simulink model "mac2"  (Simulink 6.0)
settings: Solver=ode45  StartTime=0.0  StopTime=2000  RelTol=1e-3
undefined symbols (not defined in the file or in its folder): coef, data, Ft, netlist, Ts
libraries: xbsIndex_r3 x35, dspsnks4 x1

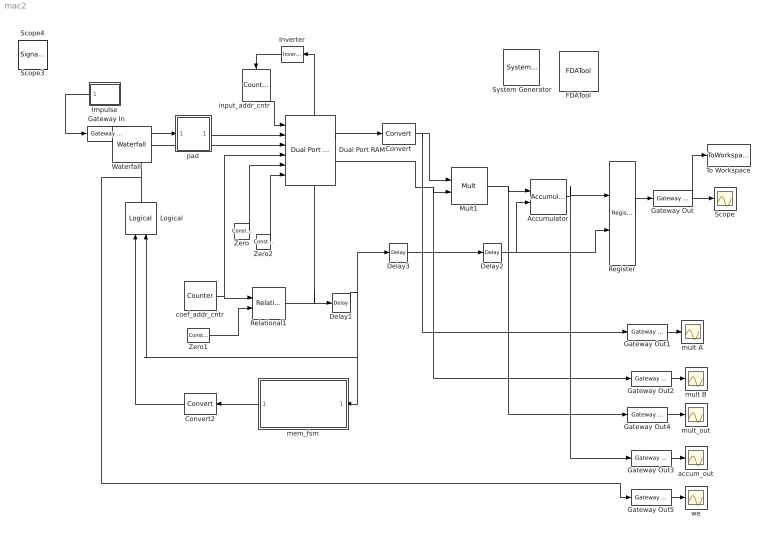
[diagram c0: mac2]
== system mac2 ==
  " System Generator" : xbsIndex_r3/ System Generator  Tag=genX  xilinxfamily=Virtex2  part=xc2v1000  speed=-4  package=fg456  synthesis_tool=XST  directory=./netlist  testbench=off  simulink_period=1/2  sysclk_period=10  incr_netlist=off  trim_vbits=Everywhere in SubSystem  dbl_ovrd=According to Block Masks  core_generation=According to Block Masks  run_coregen=off  deprecated_control=off  eval_field=0
  Accumulator : xbsIndex_r3/Accumulator  n_bits=26  overflow=Wrap  operation=Add  scale=1  explicit_period=on  period=1  rst=on  hasbypass=off  en=off  dbl_ovrd=off  show_param=off  gen_core=off  use_rpm=on
  Convert : xbsIndex_r3/Convert  arith_type=Unsigned  n_bits=8  bin_pt=6  quantization=Truncate  overflow=Wrap  latency=0  explicit_period=off  period=1  dbl_ovrd=off  show_param=off  inserted_by_tool=off  pipeline=off
  Convert2 : xbsIndex_r3/Convert  Orientation=left  arith_type=Boolean  n_bits=8  bin_pt=6  quantization=Truncate  overflow=Wrap  latency=0  explicit_period=off  period=1  dbl_ovrd=off  show_param=off  inserted_by_tool=off  pipeline=off
  Delay1 : xbsIndex_r3/Delay  latency=1  reg_retiming=off  explicit_period=off  period=1  en=off  accept_only_valid=off  init_zero=on  dbl_ovrd=off  show_param=off
  Delay2 : xbsIndex_r3/Delay  latency=3  reg_retiming=off  explicit_period=off  period=1  en=off  accept_only_valid=off  init_zero=on  dbl_ovrd=off  show_param=off
  Delay3 : xbsIndex_r3/Delay  latency=1  reg_retiming=off  explicit_period=off  period=1  en=off  accept_only_valid=off  init_zero=on  dbl_ovrd=off  show_param=off
  Dual Port RAM1 : xbsIndex_r3/Dual Port RAM  depth=length(coef)*2  initVector=[ (data) (coef)]  write_mode_A=Read After Write  write_mode_B=Read After Write  latency=1  mem_collision=off  init_zero=on  explicit_period=off  period=1  dbl_ovrd=off  rst_a=off  init_a=0  rst_b=off  init_b=0  show_param=off  distributed_mem=off  use_rpm=off  gen_core=off
  FDATool : xbsIndex_r3/FDATool
  Gateway In : xbsIndex_r3/Gateway In  arith_type=Unsigned  n_bits=8  bin_pt=6  quantization=Truncate  overflow=Wrap  period=1  timing_constraint=None  locs_specified=off  LOCs={}  needs_fixed_name=off  dbl_ovrd=off  show_param=off
  Gateway Out{,1..5} (6 alike) : xbsIndex_r3/Gateway Out  output_type=Double  nbits=8  bin_pt=6  arith_type=Boolean  quantization=Truncate  overflow=Wrap  hdl_port=on  timing_constraint=None  locs_specified=off  LOCs={}  needs_fixed_name=off  show_param=off
  Impulse : Subsystem  Orientation=left
  Inverter : xbsIndex_r3/Inverter  Orientation=left  latency=0  explicit_period=off  period=1  en=off  dbl_ovrd=off  show_param=off
  Logical : xbsIndex_r3/Logical  Orientation=up  logical_function=AND  inputs=2  precision=Full  arith_type=Unsigned  n_bits=0  bin_pt=0  align_bp=on  latency=0  explicit_period=off  period=1  en=off  dbl_ovrd=off  show_param=off
  Mult1 : xbsIndex_r3/Mult  precision=User Defined  arith_type="Signed  (2's comp)"  n_bits=26  bin_pt=17  quantization=Truncate  overflow=Wrap  latency=3  explicit_period=off  period=1  en=off  dbl_ovrd=off  show_param=off  mult_type=Parallel  oversample=2  use_embedded=off  pipeline=on  use_rpm=on  placement_style=Rectangular Shape  gen_core=off
  Register : xbsIndex_r3/Register  init=0  reg_only_valid=on  explicit_period=off  period=1  rst=off  en=on  out_en=off  dbl_ovrd=off  show_param=off
  Relational1 : xbsIndex_r3/Relational  mode=a=b  latency=0  explicit_period=on  period=-1  en=off  dbl_ovrd=off  show_param=off
  Scope : Scope
  To Workspace : ToWorkspace  VariableName=simout  SampleTime=-1  SaveFormat=Array
  Zero : xbsIndex_r3/Constant  Priority=5  const=0  equ=P=C  arith_type="Signed  (2's comp)"  n_bits=12  bin_pt=11  opselect=C  inp2=PCIN>>17  opr=+  inp1=P  carry=CIN  iostate=0  explicit_period=on  period=1  dbl_ovrd=off
  Zero1 : xbsIndex_r3/Constant  Priority=5  const=63  equ=P=C  arith_type=Unsigned  n_bits=2*log2(length(coef))  bin_pt=0  opselect=C  inp2=PCIN>>17  opr=+  inp1=P  carry=CIN  iostate=0  explicit_period=off  period=1  dbl_ovrd=off
  Zero2 : xbsIndex_r3/Constant  Priority=5  const=0  equ=P=C  arith_type=Boolean  n_bits=12  bin_pt=11  opselect=C  inp2=PCIN>>17  opr=+  inp1=P  carry=CIN  iostate=0  explicit_period=off  period=1/8000  dbl_ovrd=off
  accum_out : Scope
  coef_addr_cntr : xbsIndex_r3/Counter  Priority=5  cnt_type=Count Limited  n_bits=ceil(log2(2*length(coef)))  bin_pt=0  arith_type=Unsigned  start_count=32  cnt_to=63  cnt_by_val=1  operation=Up  explicit_period=off  period=1  load_pin=off  rst=off  en=off  dbl_ovrd=off  show_param=off  use_rpm=on  gen_core=on
  input_addr_cntr : xbsIndex_r3/Counter  Orientation=down  Priority=5  cnt_type=Count Limited  n_bits=ceil(log2(2*length(coef)))  bin_pt=0  arith_type=Unsigned  start_count=0  cnt_to=31  cnt_by_val=1  operation=Up  explicit_period=off  period=1/8000  load_pin=off  rst=off  en=on  dbl_ovrd=off  show_param=off  use_rpm=on  gen_core=on
  mem_fsm : Subsystem  Orientation=left
  mult A : Scope
  mult B : Scope
  mult_out : Scope
  pad : Subsystem
  we : Scope
  Scope3 : SignalViewerScope  IOType=viewer  RefreshTime=0.035000
  Scope4 : SignalViewerScope  IOType=viewer  RefreshTime=0.035000
  Waterfall : dspsnks4/Waterfall  IOType=viewer  TraceProperties=off  NumTraces=6  CMapStr=autumn  TNewest=1  TOldest=0  HistoryLength=10  HistoryFull=Overwrite  UpdateInterval=1  ExportMode=Selected  MLExportName=ExportData  AutoExport=off  DisplayProperties=off  MouseMode=Orbit  AxisGrid=on  Snapshot=off  Suspend=off  SyncSnapshots=off  OpenScopeAtSimStart=off  FigPos=[243 195 405 320]  CameraView=[69.4600750684385 564.426060114276 -133.474523953492 0 18.5 3.5 0.616338299486424 -7.9078811427274 1.98411164834144 2.40985953613679 1 18.5 3]  InportDimsHint=[32 1]  AxisProperties=off  AxisColor='w'  XLabel=Amplitude  YLabel=Samples  ZLabel=Time  TriggerProperties=off  TrigStartMode=Immediately  TrigStartT=0  TrigStartN=0  TrigStartFcn=trigbegin  TrigStopMode=Never  TrigStopT=0.1  TrigStopN=1  TrigStopFcn=trigend  TrigRearmMode=Never  TrigRearmT=0  TrigRearmN=0  TrigRearmFcn=trigrearm  XformProperties=on  XformMode=None  XformFcn=abs  XformExpr=(u+1)/2
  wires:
  Gateway Out/1 -> Scope/1, To Workspace/1
  Impulse/1(Out1) -> Gateway In/1
  Mult1/1 -> Accumulator/1, Gateway Out4/1
  Zero1/1 -> Relational1/2
  input_addr_cntr/1 -> Dual Port RAM1/1
  Dual Port RAM1/2 -> Mult1/2, Gateway Out2/1
  Inverter/1 -> input_addr_cntr/1
  Zero/1 -> Dual Port RAM1/5
  Zero2/1 -> Dual Port RAM1/6
  Delay2/1 -> Accumulator/2, Register/2
  Delay3/1 -> Delay2/1
  Relational1/1 -> Inverter/1, Delay1/1
  Accumulator/1 -> Register/1, Gateway Out3/1
  Register/1 -> Gateway Out/1
  Dual Port RAM1/1 -> Convert/1
  Convert/1 -> Mult1/1, Gateway Out1/1
  Gateway Out1/1 -> mult A/1
  Gateway Out2/1 -> mult B/1
  Gateway Out4/1 -> mult_out/1
  Delay1/1 -> Delay3/1, Logical/2, mem_fsm/1(fsm_cntr_in)
  mem_fsm/1(fsm_we_out) -> Convert2/1
  Logical/1 -> Dual Port RAM1/3, Gateway Out5/1
  Convert2/1 -> Logical/1
  coef_addr_cntr/1 -> Relational1/1, Dual Port RAM1/4
  pad/1(Out1) -> Dual Port RAM1/2
  Gateway In/1 -> pad/1(In1)
  Gateway Out5/1 -> we/1
  Gateway Out3/1 -> accum_out/1

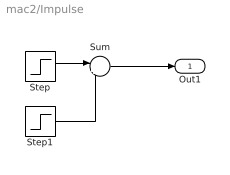
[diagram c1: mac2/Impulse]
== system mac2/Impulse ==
  Step : Step  Time=1*Ts  SampleTime=Ts
  Step1 : Step  Time=2*Ts  SampleTime=Ts
  Sum : Sum  Inputs=|+-
  Out1 : Outport
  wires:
  Step/1 -> Sum/1
  Sum/1 -> Out1/1
  Step1/1 -> Sum/2

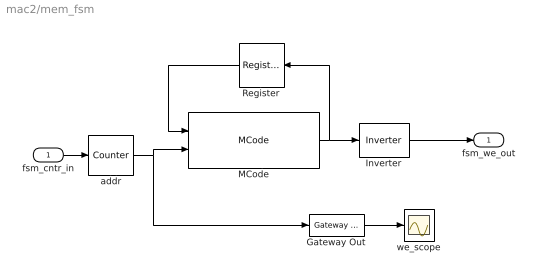
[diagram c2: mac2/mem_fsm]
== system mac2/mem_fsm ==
  fsm_cntr_in : Inport  Port=1  LatchInput=off
  Gateway Out : xbsIndex_r3/Gateway Out  output_type=Double  nbits=8  bin_pt=6  arith_type=Boolean  quantization=Truncate  overflow=Wrap  hdl_port=on  timing_constraint=None  locs_specified=off  LOCs={}  needs_fixed_name=off  show_param=off
  Inverter : xbsIndex_r3/Inverter  latency=0  explicit_period=off  period=1  en=off  dbl_ovrd=off  show_param=off
  MCode : xbsIndex_r3/MCode  mfname=lab2_fsm  defparams={}  suppress_output=off  hide_port_list={}  explicit_period=on  period=1  dbl_ovrd=off  show_param=off
  Register : xbsIndex_r3/Register  Orientation=left  init=0  reg_only_valid=off  explicit_period=on  period=1  rst=off  en=off  out_en=off  dbl_ovrd=off  show_param=off
  addr : xbsIndex_r3/Counter  Priority=5  cnt_type=Count Limited  n_bits=6  bin_pt=0  arith_type=Unsigned  start_count=0  cnt_to=32  cnt_by_val=1  operation=Up  explicit_period=off  period=1  load_pin=off  rst=off  en=on  dbl_ovrd=off  show_param=off  use_rpm=on  gen_core=on
  we_scope : Scope
  fsm_we_out : Outport
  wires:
  MCode/1 -> Register/1, Inverter/1
  Register/1 -> MCode/1
  addr/1 -> MCode/2, Gateway Out/1
  Inverter/1 -> fsm_we_out/1
  fsm_cntr_in/1 -> addr/1
  Gateway Out/1 -> we_scope/1

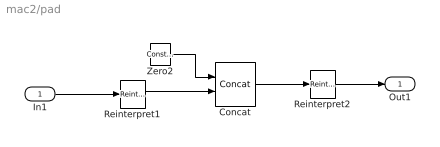
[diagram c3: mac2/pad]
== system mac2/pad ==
  In1 : Inport  Port=1  LatchInput=off
  Concat : xbsIndex_r3/Concat  num_inputs=2  explicit_period=off  period=1  dbl_ovrd=off
  Reinterpret1 : xbsIndex_r3/Reinterpret  force_arith_type=on  arith_type=Unsigned  force_bin_pt=on  bin_pt=0  force_valid=off
  Reinterpret2 : xbsIndex_r3/Reinterpret  force_arith_type=on  arith_type="Signed  (2's comp)"  force_bin_pt=on  bin_pt=11  force_valid=off
  Zero2 : xbsIndex_r3/Constant  Priority=5  const=0  equ=P=C  arith_type=Unsigned  n_bits=12-8  bin_pt=0  opselect=C  inp2=PCIN>>17  opr=+  inp1=P  carry=CIN  iostate=0  explicit_period=off  period=Ft/length(coef)  dbl_ovrd=off
  Out1 : Outport
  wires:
  Zero2/1 -> Concat/1
  In1/1 -> Reinterpret1/1
  Concat/1 -> Reinterpret2/1
  Reinterpret2/1 -> Out1/1
  Reinterpret1/1 -> Concat/2
